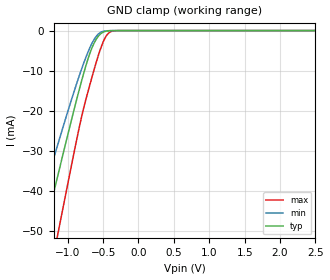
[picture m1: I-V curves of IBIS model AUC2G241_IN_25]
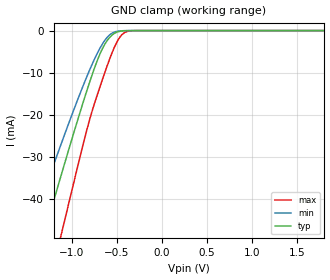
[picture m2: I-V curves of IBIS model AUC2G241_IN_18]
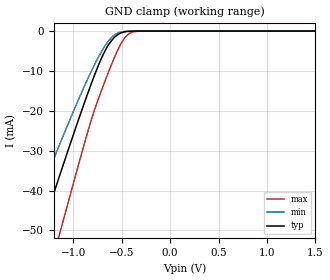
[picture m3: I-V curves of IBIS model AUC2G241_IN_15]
| TEXAS INSTRUMENTS INCORPORATED
| Standard Linear and Logic Group
| IBIS Model of SN74AUC2G241
| Dual Buffer/Driver With 3-State Outputs
| This file contains package information for the following:
|  TSSOP 8-pin (DCT) package as [Component] AUC2G241_DCT
|  TSSOP 8-pin (DCU) package as [Component] AUC2G241_DCU
|  NanoStar WCSP 8-pin (YEP) package as [Component] AUC2G241_YEP
|  NanoFree WCSP 8-pin (YZP) package as [Component] AUC2G241_YZP
| This device can be powered at the following Vccs:
|  2.5 volt Vcc
|  1.8 volt Vcc
|  1.5 volt Vcc
|  1.2 volt Vcc
|  0.8 volt Vcc
| This file provides unique models under the [Model Selector] for each Vcc.
| For operation at a specific Vcc, select the appropriate model after each
| [Model Selector] keyword.
[IBIS Ver]   3.2
[Comment char]  |_char
[File Name]   sn74auc2g241.ibs
[File Rev]   1.2 | x_die
[Date]   February 03, 2004
[Source]   Data created from TI-SPICE simulations at TI-SLL.
[Notes]   The following is an IBIS list for the AUC2G241.
   Please contact sllibis@ti.com with questions and
   comments concerning SLL IBIS models.
   - FILE REV HISTORY
   - 1.2 added YEP and YZP packages 02/03/04
   - Power clamp data deleted as there is no power-clamp diode.
   - End point warning due to AC and DC mismatch.
   - Non-monotonic data in pullup and pulldown due to
   feedback circuit.
[Disclaimer] Property of Texas Instruments Incorporated.  Unauthorized
   reproduction and/or distribution is strictly prohibited.
   This product is protected under copyright law.
   Created  2003, (C) Copyright  2003, Texas Instruments
   Incorporated, All Rights Reserved
   UNLESS THERE IS A SIGNED, WRITTEN AGREEMENT TO THE
   CONTRARY, TEXAS INSTRUMENTS (TI) IS PROVIDING THE IBIS
   MODELS  AND WITHOUT ANY WARRANTY, EXPRESSED OR
   IMPLIED.  TI assumes no liability for:
   1) the accuracy of the IBIS models provided to your
   company;
   2) the proper functioning of these IBIS Models in your
   design or for any resulting applications; or
   3) infringement of patents, copyrights or intellectual
   property rights resulting from your use of these IBIS
   models.
   TI provides IBIS Models as a service to our customers.
   You and your company shall not distribute, sell or give
   these models to anyone else without prior written
   permission from TI.
   TI reserves the right to make changes to our products or
   to discontinue any semiconductor product or service
   without notice, and advises our customers to obtain the
   latest version of relevant information to verify, before
   placing orders, that the information being relied on is
   current.
   Please be aware that your receipt and use of the IBIS
   information provided shall serve as acceptance of these
   terms and conditions.  If you do not accept these terms,
   you should return or destroy the IBIS models and any
   other accompanying information immediately.
| Component AUC2G241_DCT 8-pin TSSOP
[Component]   AUC2G241_DCT
[Manufacturer]   Texas Instruments, Inc.
[Package]
|   typ   min   max
R_pkg   2.900e-02   2.800e-02   3.100e-02
L_pkg   1.796e-09   1.666e-09   1.924e-09
C_pkg   1.090e-13   8.300e-14   1.360e-13
[Pin]   signal_name   model_name   R_pin   L_pin   C_pin
1   1NOE   AUC2G241_IN_NOE   3.100e-02   1.894e-09   1.340e-13
2   1A   AUC2G241_IN   2.800e-02   1.697e-09   8.600e-14
3   2Y   AUC2G241_OUT   3.000e-02   1.722e-09   8.600e-14
4   GND   GND   3.000e-02   1.861e-09   1.300e-13
5   2A   AUC2G241_IN   2.800e-02   1.924e-09   1.360e-13
6   1Y   AUC2G241_OUT   2.900e-02   1.736e-09   8.600e-14
7   2OE   AUC2G241_IN_OE   2.800e-02   1.666e-09   8.300e-14
8   VCC   POWER   3.000e-02   1.871e-09   1.320e-13
| Component AUC2G241_DCU 8-pin TSSOP
[Component]   AUC2G241_DCU
[Manufacturer]   Texas Instruments, Inc.
[Package]
|   typ   min   max
R_pkg   1.400e-02   1.300e-02   1.500e-02
L_pkg   1.289e-09   1.025e-09   2.014e-09
C_pkg   1.360e-13   6.600e-14   2.940e-13
[Pin]   signal_name   model_name   R_pin   L_pin   C_pin
1   1NOE   AUC2G241_IN_NOE   1.400e-02   1.387e-09   1.760e-13
2   1A   AUC2G241_IN   1.300e-02   1.026e-09   6.600e-14
3   2Y   AUC2G241_OUT   1.300e-02   1.032e-09   6.700e-14
4   GND   GND   1.500e-02   2.014e-09   2.940e-13
5   2A   AUC2G241_IN   1.400e-02   1.412e-09   1.780e-13
6   1Y   AUC2G241_OUT   1.300e-02   1.030e-09   6.600e-14
7   2OE   AUC2G241_IN_OE   1.300e-02   1.025e-09   6.600e-14
8   VCC   POWER   1.400e-02   1.386e-09   1.760e-13
| Component AUC2G241_YEP 8-pin NanoStar WCSP
[Component]   AUC2G241_YEP
[Manufacturer]   Texas Instruments, Inc.
[Package]
|   typ   min   max
R_pkg   0.001   0.001   0.001
L_pkg   0.021nH   0.021nH   0.021nH
C_pkg   0.043pF   0.042pF   0.044pF
[Pin]   signal_name   model_name   R_pin   L_pin   C_pin
1   1NOE   AUC2G241_IN_NOE   0.046   2.861nH   0.321pF
2   1A   AUC2G241_IN   0.037   2.437nH   0.286pF
3   2Y   AUC2G241_OUT   0.034   2.419nH   0.286pF
4   GND   GND   0.043   2.784nH   0.321pF
5   2A   AUC2G241_IN   0.043   2.784nH   0.321pF
6   1Y   AUC2G241_OUT   0.035   2.420nH   0.286pF
7   2OE   AUC2G241_IN_OE   0.037   2.437nH   0.286pF
8   VCC   POWER   0.046   2.860nH   0.321pF
| Component AUC2G241_YZP 8-pin NanoFree WCSP
[Component]   AUC2G241_YZP
[Manufacturer]   Texas Instruments, Inc.
[Package]
|   typ   min   max
R_pkg   0.001   0.001   0.001
L_pkg   0.021nH   0.021nH   0.021nH
C_pkg   0.043pF   0.042pF   0.044pF
[Pin]   signal_name   model_name   R_pin   L_pin   C_pin
1   1NOE   AUC2G241_IN_NOE   0.046   2.861nH   0.321pF
2   1A   AUC2G241_IN   0.037   2.437nH   0.286pF
3   2Y   AUC2G241_OUT   0.034   2.419nH   0.286pF
4   GND   GND   0.043   2.784nH   0.321pF
5   2A   AUC2G241_IN   0.043   2.784nH   0.321pF
6   1Y   AUC2G241_OUT   0.035   2.420nH   0.286pF
7   2OE   AUC2G241_IN_OE   0.037   2.437nH   0.286pF
8   VCC   POWER   0.046   2.860nH   0.321pF
| Model AUC2G241_IN
[Model Selector]   AUC2G241_IN
AUC2G241_IN_25   2.5 volt Vcc
AUC2G241_IN_18   1.8 volt Vcc
AUC2G241_IN_15   1.5 volt Vcc
AUC2G241_IN_12   1.2 volt Vcc
AUC2G241_IN_08   0.8 volt Vcc
| Model AUC2G241_IN_NOE
[Model Selector]   AUC2G241_IN_NOE
AUC2G241_IN_NOE_25   2.5 volt Vcc
AUC2G241_IN_NOE_18   1.8 volt Vcc
AUC2G241_IN_NOE_15   1.5 volt Vcc
AUC2G241_IN_NOE_12   1.2 volt Vcc
AUC2G241_IN_NOE_08   0.8 volt Vcc
| Model AUC2G241_IN_OE
[Model Selector]   AUC2G241_IN_OE
AUC2G241_IN_OE_25   2.5 volt Vcc
AUC2G241_IN_OE_18   1.8 volt Vcc
AUC2G241_IN_OE_15   1.5 volt Vcc
AUC2G241_IN_OE_12   1.2 volt Vcc
AUC2G241_IN_OE_08   0.8 volt Vcc
| Model AUC2G241_OUT
[Model Selector]   AUC2G241_OUT
AUC2G241_OUT_25   2.5 volt Vcc
AUC2G241_OUT_18   1.8 volt Vcc
AUC2G241_OUT_15   1.5 volt Vcc
AUC2G241_OUT_12   1.2 volt Vcc
AUC2G241_OUT_08   0.8 volt Vcc
| Models and submodels in the file (20): AUC2G241_IN_25 (Input), AUC2G241_IN_18 (Input), AUC2G241_IN_15 (Input), AUC2G241_IN_12 (Input), AUC2G241_IN_08 (Input), AUC2G241_IN_NOE_25 (Input), AUC2G241_IN_NOE_18 (Input), AUC2G241_IN_NOE_15 (Input), AUC2G241_IN_NOE_12 (Input), AUC2G241_IN_NOE_08 (Input), AUC2G241_IN_OE_25 (Input), AUC2G241_IN_OE_18 (Input), AUC2G241_IN_OE_15 (Input), AUC2G241_IN_OE_12 (Input), AUC2G241_IN_OE_08 (Input), AUC2G241_OUT_25 (3-state), AUC2G241_OUT_18 (3-state), AUC2G241_OUT_15 (3-state), AUC2G241_OUT_12 (3-state), AUC2G241_OUT_08 (3-state)
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[Model]   AUC2G241_IN_25
Model_type  Input
Vinl=0.7
Vinh=1.7
| variable   typ   min   max
C_comp   2.25pF   1.80pF   2.70pF
[Temperature Range]   40   100   -40
| Ambient temperature   25   85   -40
[Voltage range]   2.5   2.3   2.7
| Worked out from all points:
|   GND clamp passes 1 mA (typ) near -0.55 V on its own axis
[GND Clamp]
| AUC2G241_IN_25
|   Voltage   I(typ)   I(min)   I(max)
-3.6V     -222.3mA   -186mA     -267.4mA
-1.49V    -62.27mA   -49.76mA   -82.08mA
-1.35V    -51.78mA   -41.12mA   -69.61mA
-1.305V   -48.43mA   -38.37mA   -65.59mA
-1.17V    -38.45mA   -30.23mA   -53.54mA
-1.12V    -34.78mA   -27.27mA   -49.07mA
-735mV    -8.323mA   -6.326mA   -16.67mA
-635mV    -3.426mA   -2.469mA   -10.25mA
-525mV    -682.5uA   -360.1uA   -4.021mA
-430mV    -73.19uA   -34.72uA   -776.9uA
-325mV    -3.339uA   -2.005uA   -30.74uA
2.5V      313.9pA    400.8pA    470.4pA
[Model]   AUC2G241_IN_18
Model_type  Input
Vinl=0.5775
Vinh=1.2675
| variable   typ   min   max
C_comp   2.32pF   1.89pF   2.71pF
[Temperature Range]   40   100   -40
| Ambient temperature   25   85   -40
[Voltage range]   1.8   1.65   1.95
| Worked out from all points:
|   GND clamp passes 1 mA (typ) near -0.55 V on its own axis
[GND Clamp]
| AUC2G241_IN_18
|   Voltage   I(typ)   I(min)   I(max)
-3.6V     -222.3mA   -186mA     -267.4mA
-1.475V   -61.14mA   -48.83mA   -80.75mA
-1.43V    -57.76mA   -46.04mA   -76.74mA
-1.295V   -47.69mA   -37.76mA   -64.7mA
-1.1V     -33.32mA   -26.09mA   -47.29mA
-830mV    -14.31mA   -10.95mA   -23.64mA
-680mV    -5.361mA   -4.028mA   -13.09mA
-560mV    -1.272mA   -753.1uA   -5.827mA
-485mV    -290.6uA   -140.1uA   -2.305mA
-420mV    -55.81uA   -26.71uA   -608.5uA
-300mV    -1.501uA   -987.4nA   -11.88uA
1.8V      203.2pA    297.2pA    235.5pA
[Model]   AUC2G241_IN_15
Model_type  Input
Vinl=0.49
Vinh=1.04
| variable   typ   min   max
C_comp   2.35pF   1.94pF   2.68pF
[Temperature Range]   40   100   -40
| Ambient temperature   25   85   -40
[Voltage range]   1.5   1.4   1.6
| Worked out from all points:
|   GND clamp passes 1 mA (typ) near -0.55 V on its own axis
[GND Clamp]
| AUC2G241_IN_15
|   Voltage   I(typ)   I(min)   I(max)
-3.6V     -222.3mA   -186mA     -267.4mA
-1.505V   -63.39mA   -50.69mA   -83.42mA
-1.325V   -49.92mA   -39.59mA   -67.38mA
-1.17V    -38.45mA   -30.23mA   -53.54mA
-1.12V    -34.78mA   -27.27mA   -49.07mA
-840mV    -14.97mA   -11.47mA   -24.46mA
-695mV    -6.113mA   -4.618mA   -14.06mA
-570mV    -1.487mA   -910.9uA   -6.381mA
-495mV    -364.6uA   -178.7uA   -2.692mA
-430mV    -73.19uA   -34.72uA   -776.9uA
-280mV    -781.4nA   -556.2nA   -5.358uA
1.5V      165.9pA    258.5pA    172.1pA
